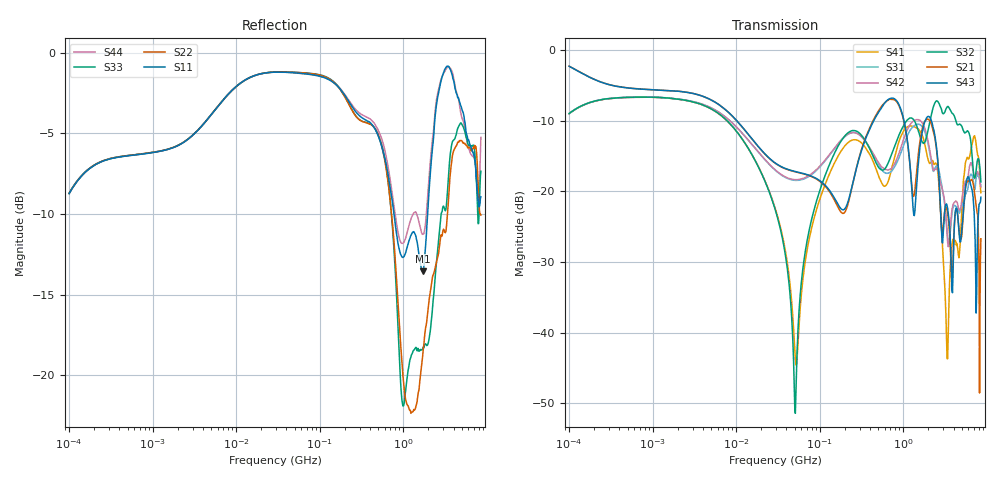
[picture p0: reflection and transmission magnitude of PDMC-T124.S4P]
# Hz S dB R 50
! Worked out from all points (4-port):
!   801 points, 100 kHz to 8.5 GHz, reference 50 ohm
!   strongest paths, dB at 100 kHz, 1.721 MHz, 29.51 MHz, 502.3 MHz, 8.5 GHz:
!     S43: -2.3, -5.7, -16.0, -8.8, -20.8
!     S21: -2.3, -5.7, -16.0, -8.6, -26.7
!     S32: -9.0, -6.8, -22.7, -16.5, -18.7
!     S42: -9.0, -6.8, -17.0, -15.8, -19.4
!     S31: -9.0, -6.8, -17.0, -16.1, -19.1
!     S41: -9.0, -6.8, -22.5, -17.7, -20.2
!   lowest |S11| = -13.6 dB at 1.711 GHz (marker M1), VSWR 1.53, Z = 76.6 + j1.12 ohm
!   |S11| at or under -10 dB: 774.1 MHz to 1.957 GHz (1.183 GHz wide, 86.6 % of centre)
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100000  -8.74 43.1  -2.25 -18.9  -8.96 -138.6  -8.97 41.5
        -2.25 -18.9  -8.73 43.1  -8.95 41.5  -8.97 -138.5
        -8.97 -138.5  -8.97 41.6  -8.71 43.1  -2.26 -18.9
        -8.97 41.5  -8.98 -138.4  -2.26 -18.9  -8.72 43.0
8898533  -2.34 15.4  -9.27 -40.4  -10.25 125.6  -10.72 -51.9
         -9.27 -40.4  -2.34 15.3  -10.71 -51.8  -10.25 125.6
         -10.25 125.6  -10.71 -51.8  -2.34 15.3  -9.26 -40.5
         -10.72 -51.9  -10.24 125.7  -9.27 -40.5  -2.34 15.3
5.109473e7  -1.25 -2.8  -17.22 -33.7  -18.43 82.7  -43.79 -30.4
            -17.22 -33.7  -1.22 -3.0  -51.45 13.1  -18.34 82.5
            -18.43 82.7  -51.42 12.9  -1.22 -3.0  -17.18 -34.4
            -43.76 -30.4  -18.33 82.5  -17.18 -34.4  -1.25 -3.0
1.717636e8  -2.20 -17.7  -22.58 -106.6  -13.05 47.3  -14.69 46.3
            -22.57 -106.5  -2.21 -20.1  -13.27 49.7  -13.02 47.4
            -13.05 47.3  -13.27 49.7  -2.19 -20.1  -22.15 -107.5
            -14.68 46.3  -13.00 47.4  -22.15 -107.5  -2.16 -17.9
1.710561e9  -13.55 1.9  -10.86 13.3  -10.95 -50.1  -12.28 -33.6
            -10.87 13.3  -18.76 -171.3  -13.09 -2.7  -10.41 -50.6
            -10.96 -50.1  -13.08 -2.6  -18.34 -124.1  -11.23 21.3
            -12.27 -33.5  -10.39 -50.6  -11.22 21.0  -11.26 -2.9
3.346927e9  -0.84 -0.4  -22.66 -31.9  -25.65 -87.9  -43.71 -18.0
            -22.64 -32.0  -10.32 37.2  -8.02 -30.4  -26.04 -84.2
            -25.64 -87.8  -8.03 -30.3  -8.96 28.8  -22.00 -29.0
            -43.68 -17.8  -26.08 -84.2  -21.99 -28.8  -0.93 8.0
8.5e9  -8.94 -4.2  -26.67 39.1  -19.05 -98.6  -20.22 43.0
       -26.70 39.9  -10.07 13.4  -18.57 -83.1  -19.41 -104.3
       -19.08 -98.3  -18.65 -83.4  -7.35 21.3  -20.71 35.6
       -20.17 43.1  -19.36 -103.5  -20.81 35.3  -5.25 2.2
